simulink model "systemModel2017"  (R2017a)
settings: Solver=VariableStepAuto  StartTime=0.0  StopTime=10.0  RelTol=1e-3
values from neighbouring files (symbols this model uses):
  c = 8e-3    (= 0.008)    [initParams.m]
  g = 9.81    [initParams.m]
  L1 = 0.5    [initParams.m]
  m = 0.2    [initParams.m]
  R = 10    [initParams.m]
  x0 = [0.1;0;0.3]    [initParams.m]

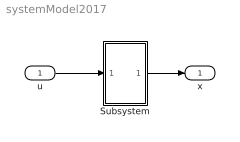
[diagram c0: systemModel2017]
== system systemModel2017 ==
  u : Inport
  Subsystem : Subsystem
  x : Outport
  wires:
  u/1 -> Subsystem/1(u)
  Subsystem/1(x) -> x/1

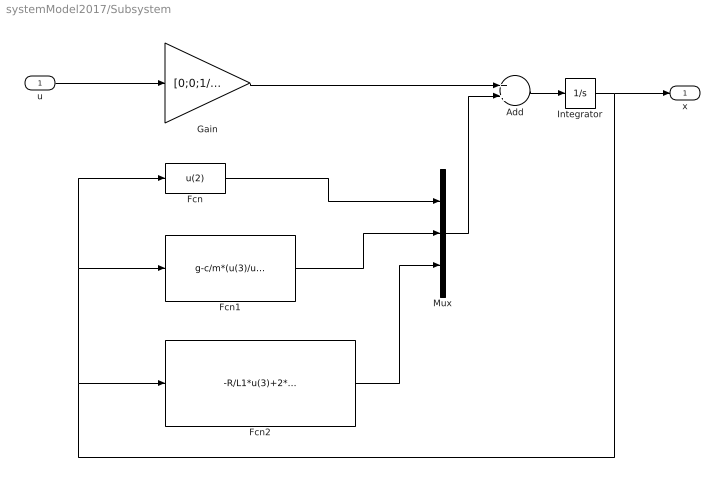
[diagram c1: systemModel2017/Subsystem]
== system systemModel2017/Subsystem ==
  u : Inport
  Add : Sum
  Fcn : Fcn  Expr=u(2)
  Fcn1 : Fcn  Expr=g-c/m*(u(3)/u(1))^2
  Fcn2 : Fcn  Expr=-R/L1*u(3)+2*c/L1*(u(2)*u(3)/(u(1))^2)
  Gain : Gain  Gain=[0;0;1/L1]  Multiplication=Matrix(K*u) (u vector)
  Integrator : Integrator  InitialCondition=x0
  Mux : Mux  Inputs=3
  x : Outport
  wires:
  Integrator/1 -> x/1, Fcn/1, Fcn1/1, Fcn2/1
  Gain/1 -> Add/1
  Fcn/1 -> Mux/1
  Fcn1/1 -> Mux/2
  Mux/1 -> Add/2
  Fcn2/1 -> Mux/3
  u/1 -> Gain/1
  Add/1 -> Integrator/1
